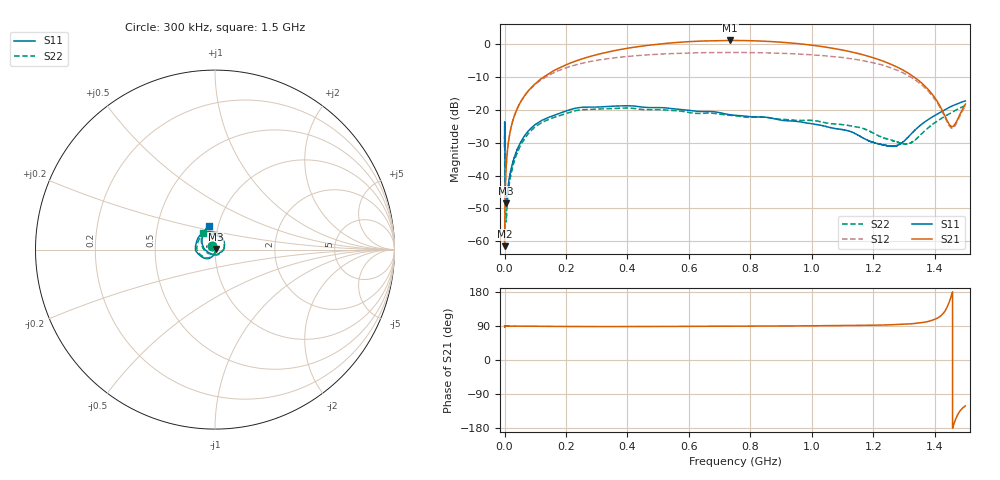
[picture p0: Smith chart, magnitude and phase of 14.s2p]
!Keysight Technologies,N5232A,MY52221221,A.10.65.11
!Date: Tuesday, May 21, 2024 18:51:08
!Correction: S11(Full 2 Port(1,4))
!S41(Full 2 Port(1,4))
!S14(Full 2 Port(1,4))
!S44(Full 2 Port(1,4))
!S2P File: Measurements: S11, S41, S14, S44:
# Hz S  RI  R 50
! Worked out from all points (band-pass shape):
!   16001 points, 300 kHz to 1.5 GHz, reference 50 ohm
!   highest |S21| = 1.10 dB at 734.4 MHz (marker M1); lowest = -61.5 dB at 300 kHz (marker M2)
!   |S21| within 3 dB of the highest: 363.0988 MHz to 363.1636 MHz (64.84 kHz wide, 0.0179 % of centre); 363.3 MHz to 1.104 GHz (740.9 MHz wide, 101 % of centre)
!   lowest |S11| = -48.5 dB at 4.705 MHz (marker M3), VSWR 1.01, Z = 50.4 + j0.0744 ohm
!   |S11| at or under -10 dB: start of sweep to end of sweep
!   |S22| runs from -54.1 to -18.7 dB; largest |S21 - S12| = 0.7
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300000  -0.0162 0.0226  1.43e-06 0.000845  -0.000794 0.000335  -0.0163 0.0208
4705369  0.0037 0.000739  0.000168 0.012  -0.0114 0.00422  0.00186 0.000827
9673125  0.00411 -0.00425  0.000295 0.0245  -0.0231 0.00884  0.00223 -0.00347
1.839013e7  0.003 -0.0104  0.000523 0.0467  -0.0432 0.0181  0.00129 -0.00905
3.348086e7  -0.000692 -0.02  0.000867 0.0845  -0.0766 0.0365  -0.00196 -0.0175
5.653875e7  -0.00967 -0.0332  0.00181 0.1422  -0.1227 0.0711  -0.0103 -0.0295
8.615782e7  -0.0254 -0.0461  0.00335 0.2156  -0.1718 0.1243  -0.0246 -0.0412
1.231817e8  -0.0476 -0.0511  0.00603 0.3056  -0.2159 0.2  -0.0442 -0.0471
2.502812e8  -0.1091 0.000503  0.0171 0.5906  -0.2281 0.4537  -0.1001 -0.00387
5.002625e8  -0.0467 0.0976  0.0263 0.9963  0.0208 0.7002  -0.0526 0.0859
7.344032e8  0.0208 0.0817  0.0161 1.134  0.278 0.6901  0.00408 0.0827
7.5015e8  0.0244 0.0789  0.0149 1.133  0.2926 0.6843  0.00773 0.0808
1.000131e9  0.0519 0.0326  -0.00407 0.9619  0.4866 0.4813  0.0456 0.0517
1.156756e9  0.0386 -0.00855  -0.0158 0.7061  0.5044 0.2658  0.0525 0.0111
1.250112e9  0.00266 -0.0282  -0.0246 0.5094  0.4303 0.1187  0.0276 -0.0222
1.281419e9  -0.0142 -0.0255  -0.0277 0.4373  0.3849 0.0789  0.0131 -0.0291
1.314318e9  -0.035 -0.0167  -0.0319 0.3588  0.328 0.0409  -0.00698 -0.0297
1.368401e9  -0.0647 0.0123  -0.0399 0.2263  0.216 0.00872  -0.0451 -0.0166
1.40655e9  -0.0727 0.0445  -0.0462 0.1305  0.131 0.0116  -0.0663 0.00585
1.453416e9  -0.064 0.0924  -0.0548 0.0122  0.0314 0.0427  -0.0765 0.0482
1.466444e9  -0.0578 0.1051  -0.0571 -0.0207  0.00588 0.0569  -0.076 0.0614
1.5e9  -0.0344 0.132  -0.0633 -0.1045  -0.0514 0.1026  -0.067 0.0945
